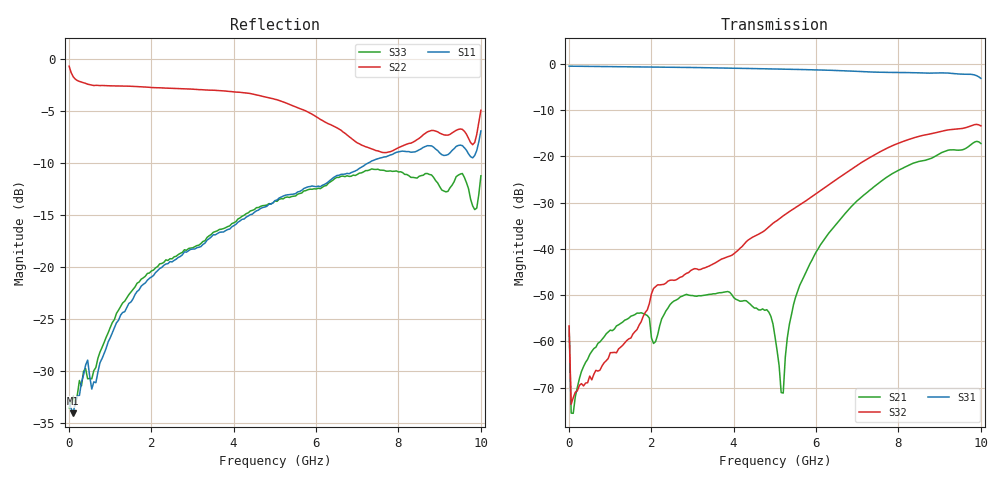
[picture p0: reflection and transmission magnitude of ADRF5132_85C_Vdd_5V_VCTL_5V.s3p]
! Device:  ADRF5132
! Description: Silicon SPDT Switch
! Frequency:  0.7 -  5 GHz
! Ports:
!	RFC	= Port 1
!	RF1	= Port 2
!  RF2  = Port 3
! Vdd:  5 Volt
! Control:  0/5 Volt
! Data:  Data was collected using a calibrated 4 port network analyzer and de-embedded using AtaiTec's In Situ De-Embedding.
! Note:  Analog Devices supplies this data as a sample of measured data
!  for this product.  Your particular data for this product may vary.
!  Data was taken at 85 degrees C.
!  Analog Devices reserves the right to change this data at anytime.
# GHZ S DB R 50.0
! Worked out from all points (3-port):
!   201 points, 10 MHz to 10 GHz, reference 50 ohm
!   strongest paths, dB at 10 MHz, 2.507 GHz, 5.005 GHz, 7.503 GHz, 10 GHz:
!     S31: -0.5, -0.7, -1.1, -1.8, -3.1
!     S32: -56.7, -46.7, -34.1, -19.2, -13.4
!     S21: -57.0, -51.6, -59.0, -25.9, -17.2
!   lowest |S11| = -34.1 dB at 109.9 MHz (marker M1), VSWR 1.04, Z = 51.9 - j0.514 ohm
!   |S11| at or under -10 dB: start of sweep to 7.266 GHz
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0.01  -33.08 -12.6  -56.89 -62.5  -0.46 -0.1
      -56.96 -60.1  -0.66 -8.2  -57.64 -60.2
      -0.46 -0.2  -56.67 -58.6  -33.56 19.5
0.1099  -34.11 -14.6  -76.14 27.6  -0.46 -1.8
        -75.57 25.3  -1.69 -69.0  -72.23 -22.0
        -0.47 -1.8  -72.19 -16.1  -32.48 -14.7
0.8092  -28.83 -74.1  -59.15 71.9  -0.52 -12.7
        -59.56 71.9  -2.52 -166.5  -65.39 -90.4
        -0.53 -12.8  -65.30 -89.9  -27.76 -65.0
3.85615  -16.40 -175.3  -49.16 68.6  -0.87 -59.3
         -49.22 68.5  -3.09 137.7  -41.69 180.0
         -0.88 -59.3  -41.70 179.9  -16.12 -123.7
5.005  -13.62 162.2  -58.94 56.7  -1.06 -76.8
       -58.99 58.4  -3.86 119.7  -34.13 176.4
       -1.08 -76.8  -34.14 176.3  -13.65 -137.8
5.2048  -13.18 158.1  -72.30 -174.0  -1.09 -79.8
        -71.19 -168.5  -4.11 117.2  -32.83 173.8
        -1.11 -79.8  -32.84 173.7  -13.45 -140.1
5.45455  -12.99 153.4  -52.07 -148.5  -1.13 -83.8
         -52.05 -148.7  -4.50 113.4  -31.32 169.4
         -1.14 -83.8  -31.32 169.3  -13.19 -143.2
6.25375  -11.95 139.1  -37.20 -169.3  -1.31 -96.6
         -37.25 -169.2  -6.12 104.6  -26.46 155.8
         -1.32 -96.6  -26.47 155.8  -12.16 -151.3
9.6004  -8.53 69.4  -18.40 65.0  -2.18 -149.9
        -18.40 65.0  -6.94 97.2  -13.82 47.4
        -2.21 -149.9  -13.83 47.3  -11.39 160.5
10  -6.90 30.0  -17.18 23.6  -3.08 -170.5
    -17.19 23.7  -4.92 26.7  -13.37 22.3
    -3.10 -170.5  -13.39 22.3  -11.23 113.0
